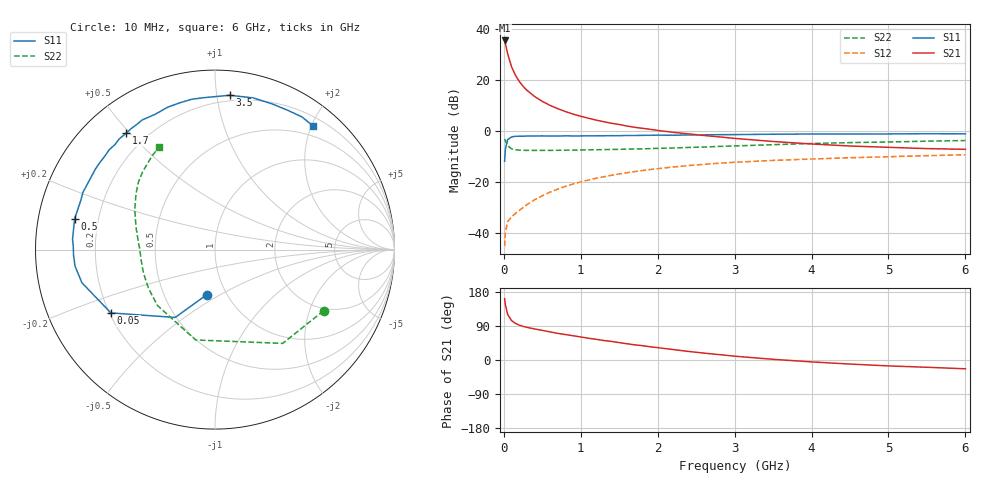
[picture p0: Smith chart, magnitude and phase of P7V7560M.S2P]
! SIEMENS Small Signal Semiconductors
! BFP196
! Si NPN RF Bipolar Junction Transistor in SOT143
! VCE = 0.75 V  IC = 60 mA
! Common Emitter S-Parameters:  May  1996
# GHz  S  MA  R  50
!  f  S11  S21  S12  S22
! GHz  MAG  ANG  MAG  ANG  MAG  ANG  MAG  ANG
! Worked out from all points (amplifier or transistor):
!   36 points, 10 MHz to 6 GHz, reference 50 ohm
!   highest |S21| = 35.5 dB at 10 MHz (marker M1)
!   |S21| within 3 dB of that: start of sweep to 33.11 MHz
!   unconditionally stable (mu >= 1): 281.7 MHz to end of sweep
!   at 250 MHz: K = 0.98, MSG = 23.8 dB, |S12| = -30.0 dB
!   at 1.4 GHz: K = 1.14, MAG = 7.9 dB, |S12| = -17.4 dB
!   at 6 GHz: K = 1.05, MAG = -0.3 dB, |S12| = -9.3 dB
!   S11 on the Smith chart (normalised r, x): 10 MHz: 0.81, -0.43; 50 MHz: 0.21, -0.27; 500 MHz: 0.11, +0.11; 1.7 GHz: 0.13, +0.49; 3.5 GHz: 0.16, +1.09; 6 GHz: 0.34, +2.03
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0.01  0.2551 -100.3  59.66 161.6  0.0055 69.9  0.6946 -29.4
0.02  0.4383 -120.4  51.74 145.9  0.0102 60.3  0.6443 -54.2
0.05  0.679 -148.7  32.51 120.1  0.0167 45.1  0.515 -102.1
0.1  0.7641 -166.0  18.22 104.0  0.0207 42.6  0.447 -135.9
0.15  0.7853 -173.3  12.45 96.7  0.0241 47.2  0.4287 -149.9
0.2  0.7889 -178.0  9.416 92.0  0.0274 52.0  0.4207 -157.7
0.25  0.7896 178.7  7.514 88.7  0.0316 55.0  0.4184 -163.0
0.3  0.7958 175.9  6.303 86.2  0.0359 57.5  0.4164 -166.1
0.4  0.7966 171.1  4.746 81.9  0.0448 60.6  0.4156 -170.9
0.5  0.8008 167.7  3.807 78.2  0.0535 62.0  0.4162 -174.1
0.6  0.7966 163.4  3.184 74.2  0.063 63.2  0.4161 -176.4
0.7  0.7966 159.7  2.742 70.3  0.0723 62.6  0.4179 -178.3
0.9  0.7994 153.0  2.142 64.0  0.0912 61.1  0.4207 178.4
1.1  0.8034 146.0  1.777 57.4  0.109 59.0  0.4266 175.8
1.3  0.8056 139.2  1.519 51.4  0.1266 56.0  0.4311 173.2
1.7  0.8157 127.2  1.18 40.0  0.1598 49.9  0.443 168.2
2.2  0.8242 114.0  0.941 27.6  0.1965 42.0  0.4635 162.1
2.8  0.8477 98.7  0.766 14.2  0.2331 32.5  0.4982 153.9
3.5  0.8637 84.6  0.622 1.8  0.2644 22.1  0.5387 144.8
4.5  0.872 68.7  0.507 -10.7  0.2985 9.8  0.5907 133.2
5.5  0.8839 56.7  0.451 -19.2  0.3278 -1.0  0.6305 123.5
6  0.879 51.5  0.437 -23.2  0.3416 -6.7  0.6501 118.6
